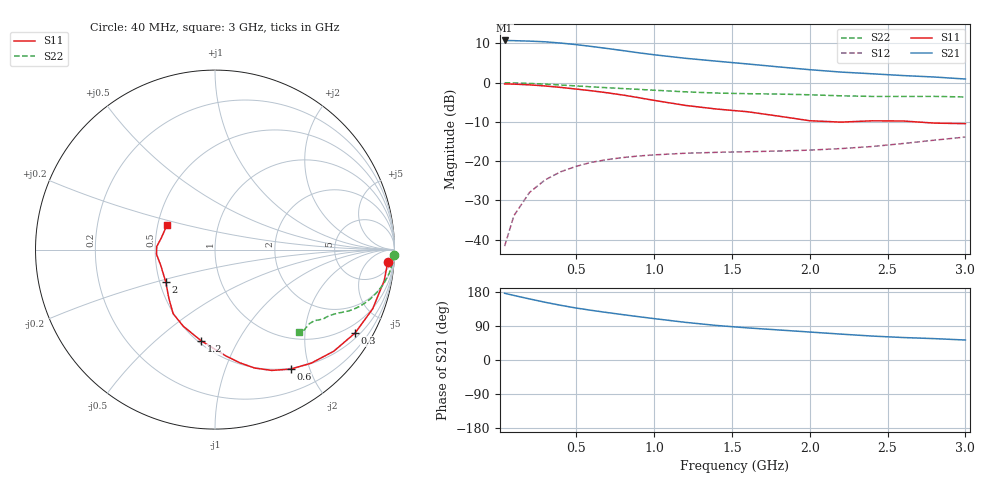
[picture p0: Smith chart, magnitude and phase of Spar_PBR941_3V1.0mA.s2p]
! Filename:  PBR941B.S2P  Version:  3.0
! NXP part #:  PBR941  Date: July 1998
! Bias condition:  Vce=3V, Ic=1.0mA
#  MHz  S  MA  R 50
! Freq  S11  S21  S12  S22
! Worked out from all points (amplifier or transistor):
!   21 points, 40 MHz to 3 GHz, reference 50 ohm
!   highest |S21| = 10.8 dB at 40 MHz (marker M1)
!   |S21| within 3 dB of that: start of sweep to 875.2 MHz
!   unconditionally stable (mu >= 1): 1.895 GHz to end of sweep
!   at 300 MHz: K = 0.18, MSG = 17.6 dB, |S12| = -24.8 dB
!   at 1 GHz: K = 0.55, MSG = 12.8 dB, |S12| = -18.4 dB
!   at 3 GHz: K = 1.07, MAG = 5.8 dB, |S12| = -13.8 dB
!   S11 on the Smith chart (normalised r, x): 40 MHz: 11, -22; 300 MHz: 0.66, -3.52; 600 MHz: 0.49, -1.71; 1.2 GHz: 0.52, -0.72; 2 GHz: 0.54, -0.22; 3 GHz: 0.56, +0.17
40  0.965 -4.1  3.449 176.1  0.008286 85.0  0.9972 -1.6
100  0.9588 -10.3  3.428 170.3  0.02031 83.9  0.9931 -4.0
200  0.9385 -20.6  3.382 161.2  0.04004 77.8  0.9789 -7.9
300  0.9084 -30.8  3.315 152.4  0.05782 72.5  0.9584 -11.5
400  0.8707 -40.6  3.194 144.4  0.07338 67.6  0.9338 -14.8
500  0.8292 -49.7  3.053 137.1  0.08609 63.7  0.9092 -17.5
600  0.7881 -57.7  2.889 130.9  0.09708 60.1  0.8848 -19.8
700  0.7437 -64.8  2.725 125.2  0.1049 57.5  0.8626 -21.7
800  0.696 -71.5  2.561 119.7  0.1114 55.5  0.8419 -23.2
900  0.645 -77.7  2.403 114.4  0.1165 53.6  0.8217 -24.5
1000  0.5956 -84.2  2.268 109.3  0.1204 52.3  0.8018 -25.6
1200  0.514 -98.6  2.046 99.4  0.1264 50.4  0.7648 -27.7
1400  0.462 -112.5  1.88 91.2  0.1297 50.0  0.7377 -29.8
1600  0.4266 -123.1  1.732 84.7  0.132 52.1  0.7243 -31.4
1800  0.3754 -133.1  1.589 79.3  0.1348 55.4  0.7165 -32.7
2000  0.3277 -147.0  1.464 73.8  0.1385 58.7  0.7014 -33.9
2200  0.3147 -163.8  1.365 68.3  0.1448 62.5  0.6808 -35.6
2400  0.3269 -175.4  1.298 63.2  0.1538 66.7  0.6686 -38.1
2600  0.3252 177.1  1.232 59.3  0.168 71.0  0.6683 -40.9
2800  0.3057 167.5  1.181 56.4  0.1853 74.4  0.6694 -42.8
3000  0.3007 152.4  1.113 52.7  0.2032 76.8  0.6574 -44.3
